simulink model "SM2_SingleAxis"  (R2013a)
settings: Solver=ode23tb  StartTime=0  StopTime=2  FixedStep=1e-4  MaxStep=0.5e-3  RelTol=1e-3  AbsTol=1e-4
PreLoadFcn:
  | warning('off','sm:sli:setup:compile:LocalSolverNotSupported')
InitFcn:
  | if(~Model.ModelUpdate)
  |  [~]=SM2_SingleAxis_ConstrFnc(0,Model);
  |  SimParam.IC = SM2_InitCondConstrFnc(RawParam,IC);
  |  Model.ModelUpdate=1;
  | end
model workspace (MAT data in the model file):
  handle : class17 (value not decoded)
  handle : class17 (value not decoded)
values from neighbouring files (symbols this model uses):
  RawParam = RobotParamGather(ParamLib)    [DeltaModelMain_v2.m]    (also in main_TimeSimulation.m; MGI.m = y)
libraries: SM2_BallJointPartsLib x2, SM2_ForeArmPartsLib x2, SM2_ArmPartsLib x1, SM2_MotorPartsLib x1, SM2_FramePartsLib x1, SM2_ToolPartsLib x1

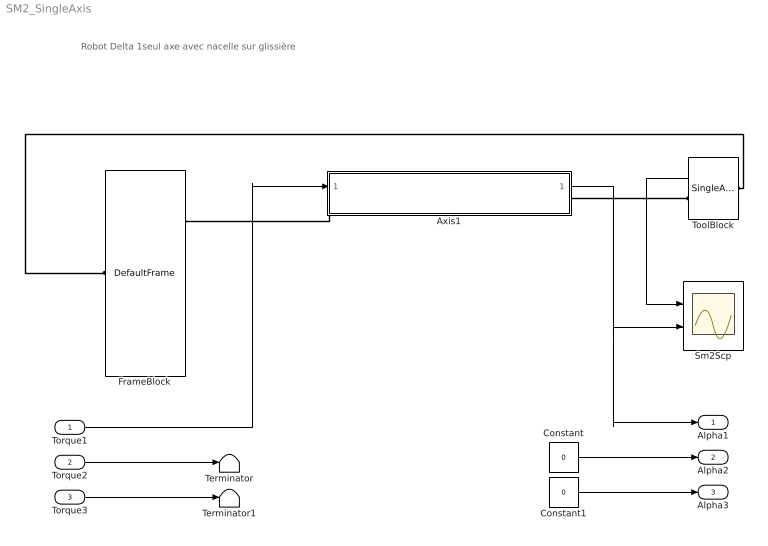
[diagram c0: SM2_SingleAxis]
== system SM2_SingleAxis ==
  note: Robot Delta 1seul axe avec nacelle sur glissière
  Torque1 : Inport
  Torque2 : Inport  Port=2
  Torque3 : Inport  Port=3
  Axis1 : Subsystem
  Constant : Constant  Value=0
  Constant1 : Constant  Value=0
  FrameBlock : SM2_FramePartsLib/DefaultFrame
  Sm2Scp : Scope  NumInputPorts=2
  Terminator : Terminator
  Terminator1 : Terminator
  ToolBlock : SM2_ToolPartsLib/SingleAxisTool
  Alpha1 : Outport
  Alpha2 : Outport  Port=2
  Alpha3 : Outport  Port=3
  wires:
  Axis1/1(Alpha) -> Sm2Scp/2, Alpha1/1
  Torque3/1 -> Terminator1/1
  Constant/1 -> Alpha2/1
  Constant1/1 -> Alpha3/1
  ToolBlock/1 -> Sm2Scp/1
  Torque2/1 -> Terminator/1
  Torque1/1 -> Axis1/1(Torque)
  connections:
  Axis1/LConn1 -- FrameBlock/RConn1
  Axis1/RConn1 -- ToolBlock/RConn1
  ToolBlock/LConn1 -- FrameBlock/LConn1

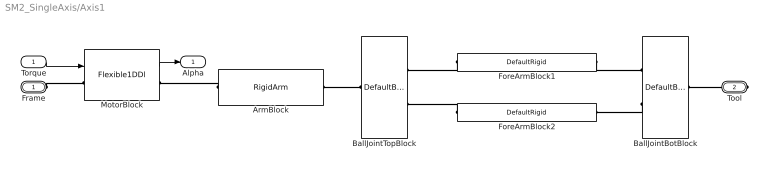
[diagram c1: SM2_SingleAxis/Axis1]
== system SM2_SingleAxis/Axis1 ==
  Torque : Inport
  ArmBlock : SM2_ArmPartsLib/RigidArm  VariantControl=armVarDefault
  BallJointBotBlock : SM2_BallJointPartsLib/DefaultBallJointBotPair
  BallJointTopBlock : SM2_BallJointPartsLib/DefaultBallJointTopPair
  ForeArmBlock1 : SM2_ForeArmPartsLib/DefaultRigid  VariantControl=foreArmVarDefault
  ForeArmBlock2 : SM2_ForeArmPartsLib/DefaultRigid  VariantControl=foreArmVarDefault
  MotorBlock : SM2_MotorPartsLib/Flexible1DDl  VariantControl=motorVarFlex1
  Frame : PMIOPort  Port=1  Side=Left
  Tool : PMIOPort  Port=2  Side=Right
  Alpha : Outport
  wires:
  Torque/1 -> MotorBlock/1
  MotorBlock/1 -> Alpha/1
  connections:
  ArmBlock/LConn1 -- MotorBlock/RConn1
  Frame/RConn1 -- MotorBlock/LConn1
  BallJointTopBlock/RConn1 -- ArmBlock/RConn1
  Tool/RConn1 -- BallJointBotBlock/RConn1
  ForeArmBlock2/LConn1 -- BallJointTopBlock/LConn2
  ForeArmBlock1/LConn1 -- BallJointTopBlock/LConn1
  ForeArmBlock1/RConn1 -- BallJointBotBlock/LConn1
  BallJointBotBlock/LConn2 -- ForeArmBlock2/RConn1
